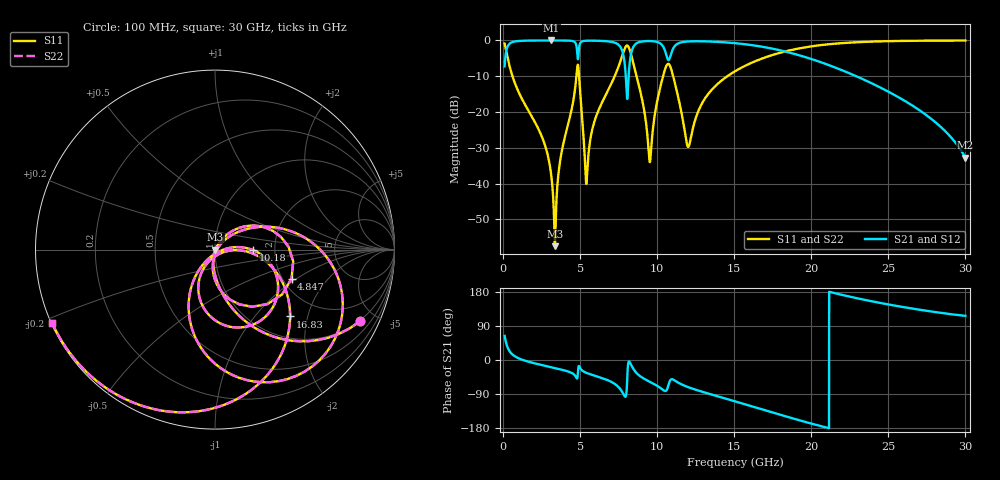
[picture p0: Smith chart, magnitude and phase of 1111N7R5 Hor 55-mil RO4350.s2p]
# GHz S MA R 50
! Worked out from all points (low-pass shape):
!   3201 points, 100 MHz to 30 GHz, reference 50 ohm
!   highest |S21| = -0.01 dB at 3.127 GHz (marker M1); lowest = -32.8 dB at 30 GHz (marker M2)
!   |S21| within 3 dB of the highest: 206.8 MHz to 4.804 GHz (4.597 GHz wide, 183 % of centre); 10.96 GHz to 18.22 GHz (7.257 GHz wide, 49.7 % of centre)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
!   lowest |S11| = -57.5 dB at 3.361 GHz (marker M3), VSWR 1.00, Z = 50.1 - j0.0633 ohm
!   |S11| at or under -10 dB: 608.7 MHz to 4.758 GHz (4.15 GHz wide, 155 % of centre); 4.929 GHz to 7.244 GHz (2.315 GHz wide, 38 % of centre); 11.04 GHz to 14.56 GHz (3.517 GHz wide, 27.5 % of centre)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
!   |S22| runs from -57.5 to 0.0 dB; largest |S21 - S12| = 0
!   S11 on the Smith chart (normalised r, x): 100 MHz: 0.96, -4.05; 4.847 GHz: 2.23, -0.91; 10.18 GHz: 1.54, -0.01; 16.83 GHz: 1.44, -1.56; 30 GHz: 0.00, -0.21
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0.1  0.9004 -26.4  0.4346 63.6  0.4346 63.6  0.9004 -26.4
0.7166875  0.2703 -78.8  0.9622 11.1  0.9622 11.1  0.2703 -78.8
3.127375  0.01294 -103.8  0.9984 -19.0  0.9984 -19.0  0.01294 -103.8
3.360969  0.001331 -28.3  0.9983 -21.2  0.9983 -21.2  0.001331 -28.3
4.846625  0.4561 -20.7  0.5549 -38.2  0.5549 -38.2  0.4561 -20.7
5.089563  0.1046 -96.8  0.9598 -26.1  0.9598 -26.1  0.1046 -96.8
5.425937  0.01107 -0.7  0.9901 -34.2  0.9901 -34.2  0.01107 -0.7
5.958531  0.07719 44.4  0.9907 -41.4  0.9907 -41.4  0.07719 44.4
7.444187  0.404 16.3  0.8851 -69.5  0.8851 -69.5  0.404 16.3
7.986125  0.8322 -36.5  0.2582 -92.7  0.2582 -92.7  0.8322 -36.5
8.481344  0.4501 -107.0  0.8295 -25.2  0.8295 -25.2  0.4501 -107.0
9.499813  0.02082 -77.4  0.9794 -57.1  0.9794 -57.1  0.02082 -77.4
10.06978  0.1666 3.6  0.9387 -69.9  0.9387 -69.9  0.1666 3.6
10.18191  0.2127 -0.8  0.913 -73.0  0.913 -73.0  0.2127 -0.8
10.83597  0.4377 -79.0  0.5841 -54.4  0.5841 -54.4  0.4377 -79.0
12.02262  0.03256 -57.8  0.9671 -71.8  0.9671 -71.8  0.03256 -57.8
13.07847  0.1516 -2.2  0.9701 -85.7  0.9701 -85.7  0.1516 -2.2
15.05  0.3704 -21.0  0.9152 -109.1  0.9152 -109.1  0.3704 -21.0
16.82531  0.5602 -41.7  0.815 -130.5  0.815 -130.5  0.5602 -41.7
20.03956  0.8275 -79.0  0.5466 -168.2  0.5466 -168.2  0.8275 -79.0
25.01978  0.9763 -124.3  0.1912 146.4  0.1912 146.4  0.9763 -124.3
30  0.9956 -155.8  0.02294 116.5  0.02294 116.5  0.9956 -155.8
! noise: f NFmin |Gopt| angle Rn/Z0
0.1  0.001388  0.8661  1.895  0.002227
3.417  0.009699  0.4754  21.5  0.003045
6.743  0.03204  0.6562  40.65  0.01572
10.06  0.09156  0.8083  60.41  0.07456
13.39  0.06073  0.6551  77.66  0.02093
16.7  0.0637  0.615  91.05  0.01599
20.03  0.08818  0.6798  104.9  0.021
23.35  0.1456  0.7874  121  0.03573
26.67  0.3125  0.8959  138.6  0.0835
30  1.504  0.9775  156.1  0.6653
